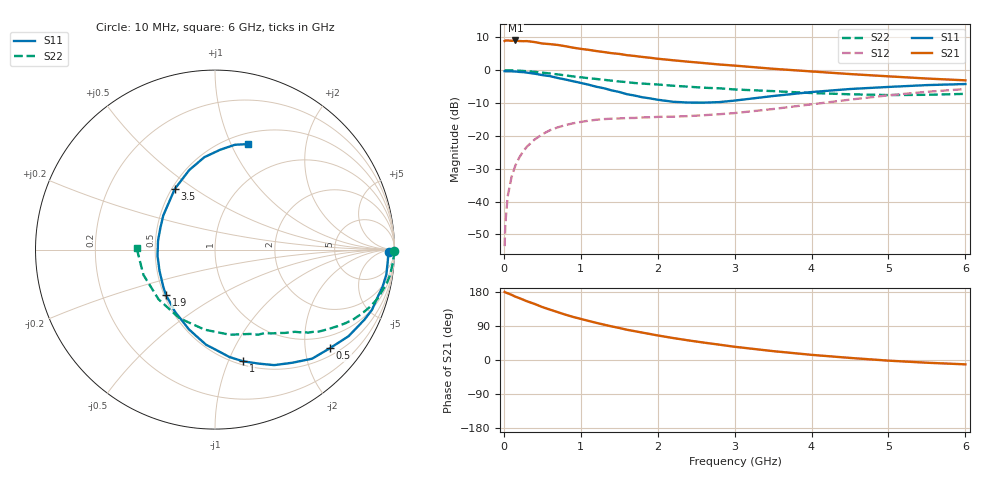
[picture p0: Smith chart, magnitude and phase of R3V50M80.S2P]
! SIEMENS Small Signal Semiconductors
! BFR181
! Si NPN RF Bipolar Junction Transistor in SOT23
! VCE = 0.5 V  IC = 0.8 mA
! Common Emitter S-Parameters:  May  1996
# GHz  S  MA  R  50
!  f  S11  S21  S12  S22
! GHz  MAG  ANG  MAG  ANG  MAG  ANG  MAG  ANG
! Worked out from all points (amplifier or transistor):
!   36 points, 10 MHz to 6 GHz, reference 50 ohm
!   highest |S21| = 9.1 dB at 150 MHz (marker M1)
!   |S21| within 3 dB of that: start of sweep to 1.142 GHz
!   unconditionally stable (mu >= 1): 1.96 GHz to 4.611 GHz
!   at 250 MHz: K = 0.15, MSG = 16.8 dB, |S12| = -24.7 dB
!   at 1.4 GHz: K = 0.76, MSG = 10.0 dB, |S12| = -14.8 dB
!   at 6 GHz: K = 0.99, MSG = 1.3 dB, |S12| = -5.7 dB
!   S11 on the Smith chart (normalised r, x): 10 MHz: 51, -21; 500 MHz: 0.67, -2.56; 1 GHz: 0.54, -1.13; 1.9 GHz: 0.51, -0.30; 3.5 GHz: 0.52, +0.42; 6 GHz: 0.61, +1.17
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0.01  0.9668 -0.8  2.789 179.6  0.0021 92.5  0.9979 -0.4
0.02  0.9657 -1.9  2.836 178.3  0.0047 85.4  0.9983 -0.9
0.05  0.9646 -4.2  2.839 176.1  0.012 86.2  0.9964 -2.2
0.1  0.9647 -8.3  2.805 172.1  0.0237 85.7  0.9935 -4.3
0.15  0.9562 -12.6  2.841 167.1  0.0355 80.3  0.9882 -6.6
0.3  0.9196 -25.1  2.776 155.0  0.0687 73.3  0.9656 -12.8
0.4  0.8872 -32.9  2.685 148.0  0.0882 67.8  0.946 -16.8
0.5  0.8443 -40.5  2.552 139.7  0.1062 63.2  0.9203 -20.3
0.7  0.7633 -55.7  2.427 126.3  0.1351 54.5  0.8647 -26.6
0.8  0.723 -62.9  2.322 119.7  0.1464 50.9  0.8349 -29.4
1  0.6418 -75.9  2.116 108.5  0.1635 44.6  0.7812 -34.1
1.1  0.6035 -82.4  2.047 103.2  0.1705 42.2  0.7584 -36.2
1.4  0.4943 -101.9  1.82 88.7  0.183 36.2  0.6951 -41.7
1.6  0.4322 -115.9  1.696 79.8  0.1874 34.1  0.6595 -44.3
1.9  0.3731 -137.0  1.55 68.6  0.1921 32.7  0.6152 -48.7
2.2  0.3313 -158.9  1.419 58.0  0.1966 32.8  0.5809 -53.1
2.6  0.3213 171.2  1.286 45.9  0.2068 34.8  0.5415 -59.1
3  0.3453 146.6  1.177 34.9  0.2228 37.0  0.51 -67.1
3.5  0.4053 123.6  1.053 23.4  0.2569 38.9  0.4812 -80.2
4.5  0.5182 96.6  0.875 5.5  0.3569 36.3  0.4307 -117.3
5.5  0.5943 79.3  0.748 -7.2  0.4696 25.2  0.4229 -160.5
6  0.6169 72.4  0.702 -11.5  0.5173 17.8  0.4369 178.9
